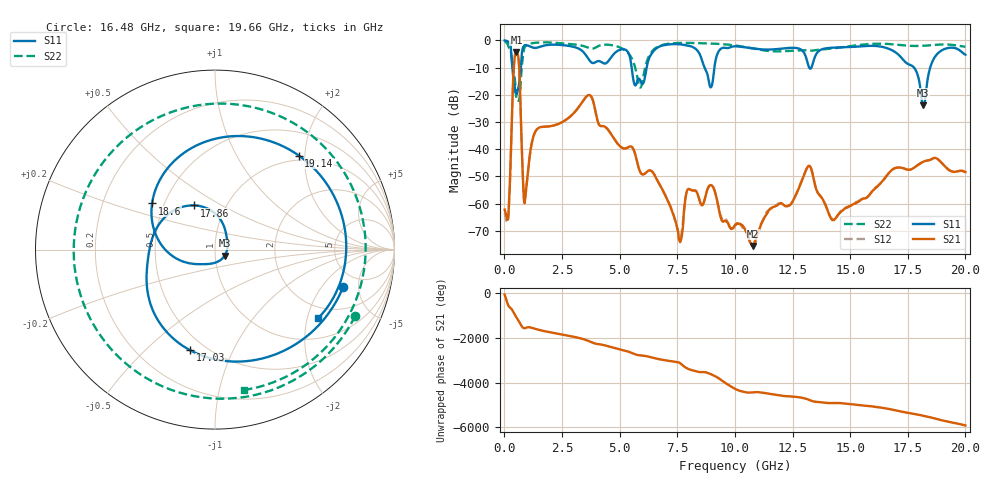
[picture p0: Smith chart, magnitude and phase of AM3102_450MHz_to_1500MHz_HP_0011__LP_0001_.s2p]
!Agilent Technologies,E8364B,MY43040894,A.07.50.67
!Agilent E8364B: A.07.50.67
!Date: Thursday, January 11, 2018 05:30:06
!Correction: S11(Full 2 Port(1,2))
!S21(Full 2 Port(1,2))
!S12(Full 2 Port(1,2))
!S22(Full 2 Port(1,2))
!S2P File: Measurements: S11, S21, S12, S22:
# Hz S  dB  R 50
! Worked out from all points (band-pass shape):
!   1601 points, 10 MHz to 20 GHz, reference 50 ohm
!   highest |S21| = -4.27 dB at 522.2 MHz (marker M1); lowest = -75.6 dB at 10.77 GHz (marker M2)
!   |S21| within 3 dB of the highest: 434.7 MHz to 620.2 MHz (185.5 MHz wide, 35.2 % of centre)
!   lowest |S11| = -23.9 dB at 18.18 GHz (marker M3), VSWR 1.14, Z = 55.5 - j3.84 ohm
!   |S11| at or under -10 dB: 5.521 GHz to 6.173 GHz (651.5 MHz wide, 11.1 % of centre); 8.684 GHz to 9.111 GHz (427.2 MHz wide, 4.8 % of centre); 17.77 GHz to 18.47 GHz (705.6 MHz wide, 3.89 % of centre)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
!   |S22| runs from -22.2 to -0.4 dB; largest |S21 - S12| = 0.0035
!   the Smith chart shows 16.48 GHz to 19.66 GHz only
!   S11 on the Smith chart (normalised r, x): 16.48 GHz: 3.58, -3.32; 17.03 GHz: 0.41, -0.69; 17.86 GHz: 0.71, +0.38; 18.6 GHz: 0.43, +0.27; 19.14 GHz: 0.91, +1.88; 19.66 GHz: 1.61, -2.34
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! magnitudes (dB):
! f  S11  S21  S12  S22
! 10 MHz  -0.1  -62.2  -63.6  -0.4
! 184.9 MHz  -0.6  -62.6  -63.3  -2.5
! 522.2 MHz  -19.0  -4.3  -4.3  -21.5
! 897.1 MHz  -1.8  -58.5  -58.5  -2.3
! 1.384 GHz  -2.8  -33.0  -33.0  -0.9
! 3.346 GHz  -3.7  -23.1  -23.1  -1.9
! 6.682 GHz  -2.5  -52.2  -52.2  -2.3
! 7.619 GHz  -1.5  -74.1  -72.3  -1.0
! 8.018 GHz  -2.0  -54.7  -54.7  -1.0
! 10.01 GHz  -2.2  -67.9  -68.0  -1.9
! 10.77 GHz  -3.0  -75.6  -75.7  -3.0
! 13.34 GHz  -9.6  -48.1  -48.0  -3.8
! 14.27 GHz  -2.7  -66.0  -65.7  -3.0
! 16.48 GHz  -2.6  -51.0  -51.0  -1.3
! 16.68 GHz  -3.1  -48.8  -48.8  -1.4
! 17.03 GHz  -4.8  -46.8  -46.8  -1.6
! 17.86 GHz  -11.3  -46.3  -46.3  -2.1
! 18.18 GHz  -23.9  -44.6  -44.7  -2.0
! 18.6 GHz  -7.2  -43.4  -43.4  -1.7
! 19.14 GHz  -3.1  -46.5  -46.5  -1.5
! 19.66 GHz  -3.2  -48.2  -48.1  -2.0
! 20 GHz  -5.3  -48.4  -48.5  -2.4
